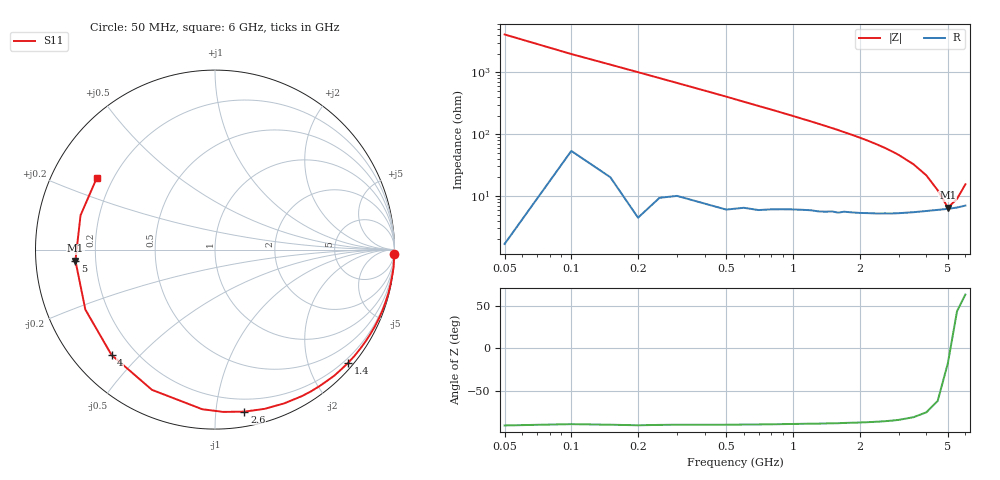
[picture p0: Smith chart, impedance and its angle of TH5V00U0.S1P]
! SIEMENS Discrete & RF Semiconductors
! BAS70
! Si Schottky Diode in SOT23
! VR = 5 V
! S-Parameters:  February  1997
# GHz  S  MA  R  50
!  f  S11
! GHz  MAG  ANG
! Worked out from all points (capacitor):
!   34 points, 50 MHz to 6 GHz, reference 50 ohm
!   read as one part to ground: C = 796 fF near 50 MHz
!   lowest |Z| = 6.48 ohm at 5 GHz (marker M1)
!   series resonance near 5.119 GHz, so ESL is about 1.2 nH
!   S11 on the Smith chart (normalised r, x): 50 MHz: 0, -82; 1.4 GHz: 0.11, -2.71; 2.6 GHz: 0.10, -1.19; 4 GHz: 0.11, -0.41; 5 GHz: 0.12, -0.04; 6 GHz: 0.14, +0.28
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0.05  1 -1.4
0.1  0.9986 -2.9
0.2  0.9996 -5.7
0.4  0.9971 -11.3
0.5  0.9964 -14.1
0.7  0.993 -19.9
0.8  0.9906 -22.7
0.9  0.9881 -25.6
1  0.9854 -28.5
1.1  0.9825 -31.5
1.2  0.9796 -34.4
1.3  0.9771 -37.4
1.4  0.9738 -40.4
1.6  0.967 -46.5
1.8  0.9576 -52.8
1.9  0.9536 -56.0
2  0.9494 -59.2
2.2  0.9396 -65.8
2.4  0.9293 -72.7
2.6  0.9175 -79.7
2.8  0.9055 -87.1
3  0.8922 -94.6
3.5  0.8567 -114.2
4  0.8226 -134.5
4.5  0.7959 -155.2
5  0.7801 -175.5
5.5  0.7731 165.7
6  0.7704 148.7
